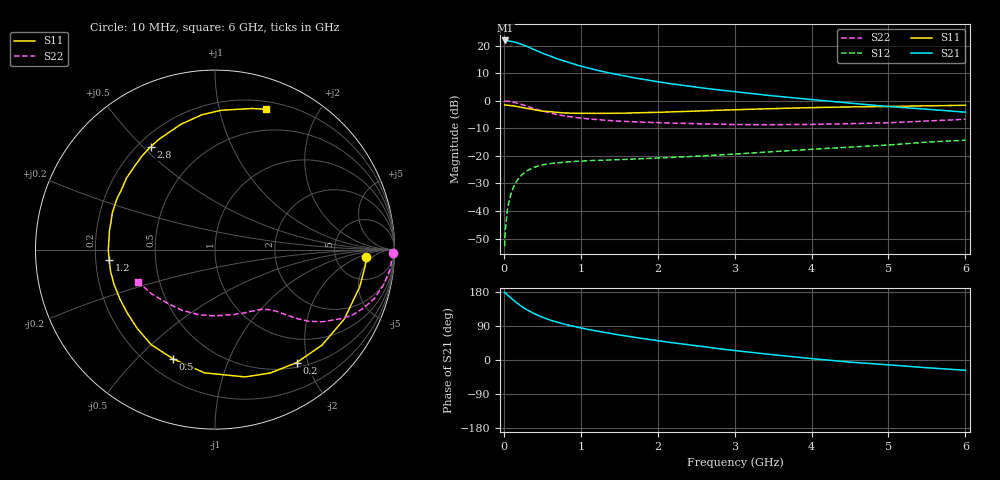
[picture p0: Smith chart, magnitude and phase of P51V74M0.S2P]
! SIEMENS Small Signal Semiconductors
! BFP183
! Si NPN RF Bipolar Junction Transistor in SOT143
! VCE = 1.75 V  IC = 4 mA
! Common Emitter S-Parameters:  March  1996
# GHz  S  MA  R  50
!  f  S11  S21  S12  S22
! GHz  MAG  ANG  MAG  ANG  MAG  ANG  MAG  ANG
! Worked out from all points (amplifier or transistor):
!   36 points, 10 MHz to 6 GHz, reference 50 ohm
!   highest |S21| = 21.9 dB at 20 MHz (marker M1)
!   |S21| within 3 dB of that: start of sweep to 368.3 MHz
!   unconditionally stable (mu >= 1): 1.658 GHz to 5.808 GHz
!   at 250 MHz: K = 0.18, MSG = 23.4 dB, |S12| = -26.5 dB
!   at 1.4 GHz: K = 0.89, MSG = 15.7 dB, |S12| = -21.4 dB
!   at 6 GHz: K = 0.97, MSG = 5.1 dB, |S12| = -14.3 dB
!   S11 on the Smith chart (normalised r, x): 10 MHz: 11, -3; 200 MHz: 0.57, -1.81; 500 MHz: 0.30, -0.64; 1.2 GHz: 0.26, -0.05; 2.8 GHz: 0.25, +0.53; 6 GHz: 0.27, +1.39
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0.01  0.8431 -2.7  12.42 178.4  0.0023 86.8  0.9944 -1.1
0.02  0.8421 -6.0  12.51 176.9  0.0046 87.9  0.986 -2.4
0.05  0.8328 -14.4  12.37 171.0  0.0116 83.6  0.9841 -5.9
0.1  0.8176 -28.3  11.96 162.3  0.0223 74.6  0.96 -11.7
0.15  0.7995 -41.7  11.59 153.7  0.0323 68.3  0.9283 -17.1
0.2  0.7764 -54.2  11.02 146.0  0.0408 62.4  0.8883 -21.6
0.25  0.7535 -65.8  10.34 138.8  0.0475 57.0  0.8459 -25.7
0.3  0.729 -76.7  9.758 132.8  0.0538 52.7  0.7976 -28.9
0.4  0.6892 -94.9  8.461 121.7  0.0626 44.7  0.7195 -34.0
0.5  0.6523 -110.9  7.355 112.9  0.0689 39.1  0.6552 -37.5
0.6  0.6378 -123.9  6.549 105.6  0.0726 35.2  0.6028 -39.8
0.7  0.6165 -134.9  5.775 99.5  0.0752 32.4  0.5608 -41.5
0.8  0.6028 -144.6  5.22 93.9  0.0773 29.8  0.5301 -42.9
1.1  0.5944 -168.1  3.946 80.4  0.0823 25.9  0.4708 -46.1
1.2  0.5929 -174.2  3.641 76.8  0.0831 25.0  0.4591 -47.2
1.7  0.6074 160.5  2.616 59.9  0.088 24.8  0.4162 -53.6
2.2  0.6339 141.1  2.023 45.3  0.0943 25.7  0.3936 -61.5
2.8  0.6756 122.1  1.579 29.7  0.1043 26.8  0.3776 -73.5
3.5  0.7236 105.2  1.233 13.9  0.1197 27.4  0.3696 -90.2
4.5  0.7769 87.5  0.911 -5.6  0.1446 24.9  0.3853 -118.6
5.5  0.8132 75.2  0.705 -20.4  0.1783 20.8  0.4304 -144.9
6  0.8319 70.0  0.624 -27.1  0.1934 17.0  0.4637 -157.0
